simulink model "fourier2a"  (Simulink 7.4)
settings: Solver=ode45  StartTime=0.0  StopTime=0.02  MaxStep=1e-5  RelTol=1e-3

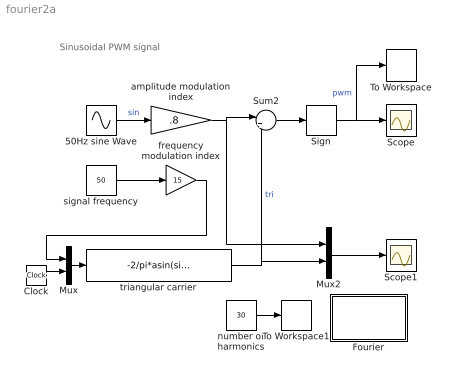
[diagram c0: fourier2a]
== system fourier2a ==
  note: Sinusoidal PWM signal
  50Hz sine Wave : Sin  Amplitude=1  Bias=0  Frequency=2*pi*50  Phase=0  Samples=10  SampleTime=0
  Clock : Clock
  Fourier : Subsystem
  Mux : Mux  Inputs=2
  Mux2 : Mux  Inputs=2
  Scope : Scope
  Scope1 : Scope
  Sign : Signum
  Sum2 : Sum  Inputs=|+-  OutDataType=sfix(16)  OutScaling=2^0
  To Workspace : ToWorkspace  VariableName=f  SampleTime=-1  SaveFormat=Array
  To Workspace1 : ToWorkspace  VariableName=h  SampleTime=-1  SaveFormat=Array
  amplitude modulation index : Gain  Gain=.8  ParameterDataType=sfix(16)  ParameterScaling=2^0  OutDataType=sfix(16)  OutScaling=2^0
  frequency modulation index : Gain  Gain=15  ParameterDataType=sfix(16)  ParameterScaling=2^0  OutDataType=sfix(16)  OutScaling=2^0
  number of harmonics : Constant  Value=30  OutDataType=sfix(16)  OutScaling=2^0
  signal frequency : Constant  Value=50  OutDataType=sfix(16)  OutScaling=2^0
  triangular carrier : Fcn  Expr=-2/pi*asin(sin(2*pi*u(1)*u(2)))
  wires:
  Sum2/1 -> Sign/1
  Sign/1 -> Scope/1, To Workspace/1  "pwm"
  50Hz sine Wave/1 -> amplitude modulation index/1  "sin"
  amplitude modulation index/1 -> Sum2/1, Mux2/1
  triangular carrier/1 -> Sum2/2, Mux2/2  "tri"
  Mux2/1 -> Scope1/1
  Mux/1 -> triangular carrier/1
  Clock/1 -> Mux/2
  signal frequency/1 -> frequency modulation index/1
  frequency modulation index/1 -> Mux/1
  number of harmonics/1 -> To Workspace1/1

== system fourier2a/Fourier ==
  note: To obtain the Fourier decomposition of a periodic signal: a) run a simulation for one period duration b) Specify the fundamental frequency c) Specify the number of harmonics
